PROGRAM MAIN
VAR
	(* 轴控变量 *)
	AxisTest                : Axis_REF;										// 测试轴
	fbAxisPower				: MC_Power;										// 使能功能块
	fbAxisMove				: MC_JOG;										// 运动功能块
	fbHalt					: MC_Halt;										// 停止功能块
	bPower					: BOOL					:= TRUE;				// 如果为TRUE，则轴使能
	bMoveFor				: BOOL;											// 如果为TRUE，轴前进
	bMoveBack				: BOOL;											// 如果为TRUE，轴后退
	
	(* 模拟升温相关变量 *)
	fbSimulater             : FB_CTRL_PT1;                                  // 模拟功能块
	stParamSimulater        : ST_CTRL_PT1_PARAMS;                           // 模拟功能块参数
	fbTimer                 : TON;                                          // 模拟温度上升前的延迟功能块
	lCurrnetTargetTemp		: LREAL     			:= 80;                  // 当前目标温度
	bActiveSimulation		: BOOL					:= FALSE;				// 如果为TRUE，模拟升温
	lActTemp				: LREAL;										// 当前实际温度
	
	(* 上升沿检测 *)
	rtProductionStart		: R_TRIG;										// 检测生产的上升沿
	rtOverTemp				: R_TRIG;										// 检测温度超过上限的上升沿							
	rtOverPositionRange		: R_TRIG;										// 检测轴超过限位的上升沿
	
	bProductionStart        : BOOL;											// 如果为TRUE，生产开始
	
	(* 消息操作变量 *)
	bMessage                : BOOL;											// 如果为TRUE，发送消息
	
	(* 报警操作变量 *)
	bAlarmCylinderTemp		: BOOL;											// 如果为TRUE，发送过温报警
	bClearCylinderTemp		: BOOL;											// 如果为TRUE，清除过温报警
	bAlarmAxisPosition		: BOOL;											// 如果为TRUE，发送轴限位报警
	bClearAxisPosition		: BOOL;											// 如果为TRUE，清除轴限位报警

	(* 导出日志 *)
	FB_EventExporter		: FB_EventExporter;								// 导出日志功能块
	bExport					: BOOL;											// 如果为TRUE，导出日志
	
END_VAR

// 延时启动
fbTimer(IN:=TRUE , PT:=T#10S , Q=> , ET=> );
IF fbTimer.Q THEN
	bProductionStart 			:= TRUE;
END_IF

EevntInstance();

Detection();

AxisMove();

SimulateTemperature();

Export();

IF rtProductionStart.Q THEN
	bMessage					:= TRUE;		// 发送消息
END_IF

IF rtOverTemp.Q THEN	
	FB_EventloggerHandlingCylinderTemp.P_TextPrefix	:= 'Cylinder1' ;
	bAlarmCylinderTemp          := TRUE;		// 发送过温报警
END_IF
	
IF rtOverPositionRange.Q THEN
	fbHalt(Axis:= AxisTest, Execute:= TRUE );	// 停止轴
	bAlarmAxisPosition          := TRUE;		// 发送轴限位报警
END_IF

ACTION AxisMove:
(* 轴控 *)
fbAxisPower(
	Axis:= AxisTest, 
	Enable:= bPower, 
	Enable_Positive:= TRUE, 
	Enable_Negative:= TRUE, 
	Override:= , 
	BufferMode:= , 
	Options:= , 
	Status=> , 
	Busy=> , 
	Active=> , 
	Error=> , 
	ErrorID=> );
	
fbAxisMove(
	Axis:= AxisTest, 
	JogForward:= bMoveFor , 
	JogBackwards:= bMoveBack, 
	Mode:= , 
	Position:= , 
	Velocity:= 300, 
	Acceleration:= , 
	Deceleration:= , 
	Jerk:= , 
	Done=> , 
	Busy=> , 
	Active=> , 
	CommandAborted=> , 
	Error=> , 
	ErrorID=> );
END_ACTION

ACTION Detection:
(* 信号上升沿检测 *)
rtOverPositionRange (CLK:= (AxisTest.NcToPlc.ActPos >= 12000));
rtOverTemp			(CLK:= (lActTemp >= 75));
rtProductionStart	(CLK:=  bProductionStart);
END_ACTION

ACTION EevntInstance:
// 调用各事件处理功能块实例
FB_EventloggerHandlingProductionInfo(bMessage := bMessage);
FB_EventloggerHandlingAxisPosition	(bAlarm   := bAlarmAxisPosition, bClear := bClearAxisPosition);
FB_EventloggerHandlingCylinderTemp	(bAlarm   := bAlarmCylinderTemp, bClear := bClearCylinderTemp);

//FB_EventloggerHandlingMyEvent(bAlarm:= , bMessage:= , bClear:= );
END_ACTION

ACTION Export:
FB_EventExporter(
	bExport:= bExport, 
	sExportFilePath:= , 
	chooseExportOption:=  , 
	EventClassID:= TC_EVENT_CLASSES.MyEvent, 
	ExportDone=> , 
	Tips=> );
END_ACTION

ACTION SimulateTemperature:
(* 设置模拟器参数 *)
stParamSimulater.fKp :=1;
stParamSimulater.tCtrlCycleTime:=T#500MS;
stParamSimulater.tTaskCycleTime:=T#10MS;
stParamSimulater.tT1:=T#20S;


(* 模拟温度 *)
IF bActiveSimulation THEN
	
   
    fbSimulater(fIn:= lCurrnetTargetTemp, eMode:=E_CTRL_MODE.eCTRL_MODE_ACTIVE , fOut=> ,  stParams:=stParamSimulater );	

	
	// 传递输出 
	lActTemp  := fbSimulater.fOut;
	
ELSE
	
	fbSimulater(eMode:=E_CTRL_MODE.eCTRL_MODE_RESET , stParams:=stParamSimulater );
END_IF
END_ACTION

END_PROGRAM
